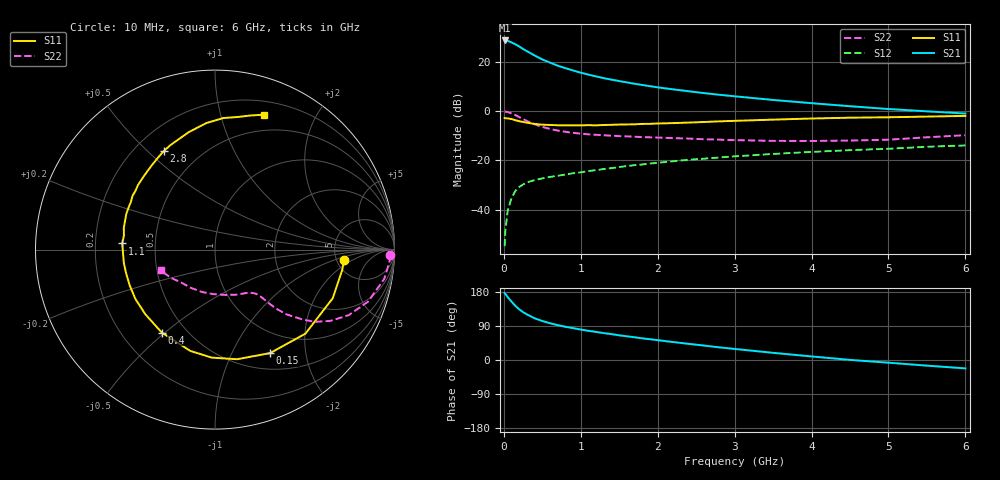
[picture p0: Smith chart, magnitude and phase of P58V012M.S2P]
! SIEMENS Small Signal Semiconductors
! BFP183
! Si NPN RF Bipolar Junction Transistor in SOT143
! VCE = 8 V  IC = 12 mA
! Common Emitter S-Parameters:  March  1996
# GHz  S  MA  R  50
!  f  S11  S21  S12  S22
! GHz  MAG  ANG  MAG  ANG  MAG  ANG  MAG  ANG
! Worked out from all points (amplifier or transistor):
!   36 points, 10 MHz to 6 GHz, reference 50 ohm
!   highest |S21| = 28.7 dB at 10 MHz (marker M1)
!   |S21| within 3 dB of that: start of sweep to 227.1 MHz
!   unconditionally stable (mu >= 1): 1.166 GHz to 5.722 GHz
!   at 250 MHz: K = 0.33, MSG = 27.5 dB, |S12| = -29.8 dB
!   at 1.4 GHz: K = 1.06, MAG = 16.5 dB, |S12| = -23.2 dB
!   at 6 GHz: K = 0.96, MSG = 6.5 dB, |S12| = -14.0 dB
!   S11 on the Smith chart (normalised r, x): 10 MHz: 5.86, -1.36; 150 MHz: 0.70, -1.42; 400 MHz: 0.37, -0.49; 1.1 GHz: 0.32, +0.03; 2.8 GHz: 0.32, +0.56; 6 GHz: 0.33, +1.37
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0.01  0.7217 -4.4  27.24 176.7  0.0018 89.5  0.9781 -1.9
0.02  0.7179 -9.1  27.23 174.5  0.0037 85.3  0.9745 -4.0
0.05  0.7098 -22.4  26.81 166.1  0.0094 82.3  0.9572 -9.8
0.1  0.6879 -42.9  24.82 153.9  0.0171 69.1  0.9006 -18.8
0.15  0.6532 -62.0  22.8 142.8  0.0238 62.1  0.83 -26.1
0.2  0.6231 -78.6  20.57 133.7  0.0288 56.9  0.7559 -31.7
0.25  0.6022 -91.7  18.26 126.3  0.0323 52.6  0.6895 -35.7
0.3  0.581 -103.7  16.52 120.3  0.0356 49.9  0.63 -38.4
0.4  0.5491 -122.7  13.47 110.1  0.0395 45.4  0.5394 -42.1
0.5  0.5296 -137.0  11.21 102.9  0.043 43.6  0.4765 -43.9
0.6  0.522 -148.1  9.666 97.0  0.046 43.0  0.4339 -44.7
0.7  0.5154 -157.2  8.37 92.1  0.0485 43.5  0.4019 -45.2
0.9  0.5133 -171.7  6.686 84.1  0.0546 43.7  0.3618 -45.9
1.1  0.5178 176.2  5.514 76.9  0.0605 44.2  0.3371 -47.0
1.3  0.5221 166.8  4.668 70.9  0.0665 44.5  0.3224 -48.7
1.6  0.5356 154.0  3.825 62.5  0.0763 44.7  0.3066 -51.9
2.2  0.5701 134.0  2.764 47.4  0.0956 42.8  0.2821 -61.6
2.8  0.6185 117.6  2.147 33.4  0.1141 39.1  0.2631 -74.3
3.5  0.6706 102.6  1.684 18.9  0.1346 34.4  0.2481 -92.3
4.5  0.7344 86.4  1.256 0.3  0.1607 26.7  0.252 -122.3
5.5  0.7737 75.0  0.989 -14.9  0.1885 19.9  0.2935 -147.9
6  0.7986 70.2  0.891 -22.1  0.2005 15.6  0.3239 -159.2
